| IBIS file stm32u535_545_ufbga64_smps.ibs
[IBIS ver] 4.2
[File name] stm32u535_545_ufbga64_smps.ibs
[File Rev] ev1.0
[Date]  11-09-2023
[Source] Data Created at STMicroelectronics
[Notes]  File originated from ELDO simulations.
[Disclaimer]  This information is for modeling purpose only and is
   not guaranteed. The information is subject to change without
   notice.
[Copyright] Copyright 2023 STMicroelectronics Inc.
|   Component stm32u535_545_ufbga64_smps
[Component] stm32u535_545_ufbga64_smps
[Manufacturer] STMicroelectronics
[Package]
| variable   typ   min   max
R_pkg  0  NA  NA
L_pkg  0  NA  NA
C_pkg  0  NA  NA
[Pin]   signal_name   model_name
A1  VDD  power
A2  VDD11  nc
A3  PH3-BOOT0  io8_100m_ft
A4  PB6  io8_100m_i2c_ft
A5  PB3  io8_100m_i2c_ft
A6  PD2  io8_100m_hslv_ft
A7  PC10  io8_100m_hslv_ft
A8  VDD  power
B1  VBAT  power
B2  VSS  gnd
B3  PC13  io8_100m_ft_v33
B4  PB4  io8_100m_i2c_ft
B5  PC11  io8_100m_hslv_ft
B6  PC12  io8_166m_hslv_ft
B7  VSS  gnd
B8  VDDUSB  power
C1  PC14-OSC32_IN   io8_100m_tamp_ft
C2  PC15-OSC32_OUT   io8_100m_tamp_ft
C3  PB8  io8_100m_hslv_i2c_ft
C4  PA15  io8_100m_ft
C5  PA14  io8_100m_ft
C6  PA13  io8_100m_ft
C7  PA12  io8_usb_ft
C8  PA11  io8_usb_ft
D1  PH0-OSC_IN  io8_100m_ft
D2  PH1-OSC_OUT  io8_100m_ft
D3  PB7  io8_166m_hslv_i2c_ft
D4  PB5  io8_166m_hslv_ft
D5  PA10  io8_100m_ft
D6  PA9  io8_100m_ft
D7  PA8  io8_166m_hslv_ft
D8  PC9  io8_100m_hslv_ft
E1  NRST  nc
E2  PC0  io8_100m_hslv_i2c_ft
E3  PC1  io8_166m_hslv_i2c_ft
E4  PC2  io8_100m_hslv_ft
E5  PA0  io8_100m_hslv_tamp_ft
E6  PB14  io8_100m_i2c_ft
E7  PC7  io8_100m_hslv_ft
E8  PC8  io8_100m_hslv_ft
F1  VSSA  nc
F2  PC3  io8_100m_hslv_ft
F3  PA1  io8_100m_hslv_tamp_ft
F4  PA4  io8_100m_hslv_ft
F5  PA6  io8_100m_hslv_ft
F6  PB10  io8_166m_hslv_i2c_ft
F7  PB15  io8_100m_ft
F8  PC6  io8_100m_hslv_ft
G1  VDDA  power
G2  PA2  io8_100m_hslv_ft
G3  PA5  io8_100m_ft
G4  PB2  io8_100m_hslv_tamp_ft
G5  PB1  io8_100m_hslv_ft
G6  VSSSMPS  nc
G7  VSS  gnd
G8  PB13  io8_100m_i2c_ft
H1  VDD  power
H2  PA3  io8_166m_hslv_ft
H3  PA7  io8_100m_hslv_i2c_ft
H4  PB0  io8_100m_hslv_ft
H5  VLXSMPS  nc
H6  VDDSMPS  nc
H7  VDD11  nc
H8  VDD  power
[Package Model]   455-ufbga-5x5-64smps-100mhz-230421
[Pin Mapping]   pulldown_ref   pullup_ref   | Comment
A1  nc  vddiom
A2  nc  nc
A3  gndio  vddiom
A4  gndio  vddiom
A5  gndio  vddiom
A6  gndio  vddiom
A7  gndio  vddiom
A8  nc  vddiom
B1  nc  vsw
B2  gndio  nc
B3  gndio  vddiom  | Depending on IO usage
| B3  gndio  vsw  | Depending on IO usage
B4  gndio  vddiom
B5  gndio  vddiom
B6  gndio  vddiom
B7  gndio  nc
B8  nc  vddusb
C1  gndio  vddiom  | Depending on IO usage
| C1  gndio  vsw  | Depending on IO usage
C2  gndio  vddiom  | Depending on IO usage
| C2  gndio  vsw  | Depending on IO usage
C3  gndio  vddiom
C4  gndio  vddiom
C5  gndio  vddiom
C6  gndio  vddiom  | Depending on IO usage
| C6  gndio  vddusb  | Depending on IO usage
C7  gndio  vddiom  | Depending on IO usage
| C7  gndio  vddusb  | Depending on IO usage
C8  gndio  vddiom  | Depending on IO usage
| C8  gndio  vddusb  | Depending on IO usage
D1  gndio  vddiom
D2  gndio  vddiom
D3  gndio  vddiom
D4  gndio  vddiom
D5  gndio  vddiom  | Depending on IO usage
| D5  gndio  vddusb  | Depending on IO usage
D6  gndio  vddiom  | Depending on IO usage
| D6  gndio  vddusb  | Depending on IO usage
D7  gndio  vddiom
D8  gndio  vddiom
E1  nc   nc
E2  gndio  vddiom
E3  gndio  vddiom
E4  gndio  vddiom
E5  gndio  vddiom
E6  gndio  vddiom
E7  gndio  vddiom
E8  gndio  vddiom
F1  nc  nc
F2  gndio  vddiom
F3  gndio  vddiom
F4  gndio  vddiom
F5  gndio  vddiom
F6  gndio  vddiom
F7  gndio  vddiom
F8  gndio  vddiom
G1  nc  vddiom
G2  gndio  vddiom
G3  gndio  vddiom
G4  gndio  vddiom
G5  gndio  vddiom
G6  nc  nc
G7  gndio  nc
G8  gndio  vddiom
H1  nc  vddiom
H2  gndio  vddiom
H3  gndio  vddiom
H4  gndio  vddiom
H5  nc  nc
H6  nc  nc
H7  nc  nc
H8  nc  vddiom
[Model Selector] io8_100m_ft
io8_100m_ft_hs_1v2  "IO8_FT 100MHz high speed @ 1.2V"
io8_100m_ft_fs_1v2  "IO8_FT 100MHz fast speed @ 1.2V"
io8_100m_ft_fs_pd_1v2  "IO8_FT 100MHz fast speed @ 1.2V pulldown"
io8_100m_ft_ms_1v2  "IO8_FT 100MHz med speed @ 1.2V"
io8_100m_ft_ms_pd_1v2  "IO8_FT 100MHz med speed @ 1.2V pulldown"
io8_100m_ft_ls_1v2  "IO8_FT 100MHz low speed @ 1.2V"
io8_100m_ft_ls_pd_1v2  "IO8_FT 100MHz low speed @ 1.2V pulldown"
io8_100m_ft_hs_1v8  "IO8_FT 100MHz high speed @ 1.8V"
io8_100m_ft_hs_pd_1v8  "IO8_FT 100MHz high speed @ 1.8V pulldown"
io8_100m_ft_fs_1v8  "IO8_FT 100MHz fast speed @ 1.8V"
io8_100m_ft_fs_pd_1v8  "IO8_FT 100MHz fast speed @ 1.8V pulldown"
io8_100m_ft_ms_1v8  "IO8_FT 100MHz med speed @ 1.8V"
io8_100m_ft_ms_pd_1v8  "IO8_FT 100MHz med speed @ 1.8V pulldown"
io8_100m_ft_ls_1v8  "IO8_FT 100MHz low speed @ 1.8V"
io8_100m_ft_ls_pd_1v8  "IO8_FT 100MHz low speed @ 1.8V pulldown"
io8_100m_ft_hs_3v3  "IO8_FT 100MHz high speed @ 3.3V"
io8_100m_ft_hs_pd_3v3  "IO8_FT 100MHz high speed @ 3.3V pulldown"
io8_100m_ft_fs_3v3  "IO8_FT 100MHz fast speed @ 3.3V"
io8_100m_ft_fs_pd_3v3  "IO8_FT 100MHz fast speed @ 3.3V pulldown"
io8_100m_ft_ms_3v3  "IO8_FT 100MHz med speed @ 3.3V"
io8_100m_ft_ms_pd_3v3  "IO8_FT 100MHz med speed @ 3.3V pulldown"
io8_100m_ft_ls_3v3  "IO8_FT 100MHz low speed @ 3.3V"
io8_100m_ft_ls_pd_3v3  "IO8_FT 100MHz low speed @ 3.3V pulldown"
[Model Selector] io8_100m_hslv_ft
io8_100m_ft_hs_1v2  "IO8_FT 100MHz high speed @ 1.2V"
io8_100m_ft_hs_pu_1v2  "IO8_FT 100MHz high speed @ 1.2V pullup"
io8_100m_ft_hs_pd_1v2  "IO8_FT 100MHz high speed @ 1.2V pulldown"
io8_100m_ft_fs_1v2  "IO8_FT 100MHz fast speed @ 1.2V"
io8_100m_ft_fs_pu_1v2  "IO8_FT 100MHz fast speed @ 1.2V pullup"
io8_100m_ft_fs_pd_1v2  "IO8_FT 100MHz fast speed @ 1.2V pulldown"
io8_100m_ft_ms_1v2  "IO8_FT 100MHz med speed @ 1.2V"
io8_100m_ft_ms_pu_1v2  "IO8_FT 100MHz med speed @ 1.2V pullup"
io8_100m_ft_ms_pd_1v2  "IO8_FT 100MHz med speed @ 1.2V pulldown"
io8_100m_ft_ls_1v2  "IO8_FT 100MHz low speed @ 1.2V"
io8_100m_ft_ls_pu_1v2  "IO8_FT 100MHz low speed @ 1.2V pullup"
io8_100m_ft_ls_pd_1v2  "IO8_FT 100MHz low speed @ 1.2V pulldown"
io8_100m_ft_hs_1v8  "IO8_FT 100MHz high speed @ 1.8V"
io8_100m_ft_hs_pu_1v8  "IO8_FT 100MHz high speed @ 1.8V pullup"
io8_100m_ft_hs_pd_1v8  "IO8_FT 100MHz high speed @ 1.8V pulldown"
io8_100m_ft_fs_1v8  "IO8_FT 100MHz fast speed @ 1.8V"
io8_100m_ft_fs_pu_1v8  "IO8_FT 100MHz fast speed @ 1.8V pullup"
io8_100m_ft_fs_pd_1v8  "IO8_FT 100MHz fast speed @ 1.8V pulldown"
io8_100m_ft_ms_1v8  "IO8_FT 100MHz med speed @ 1.8V"
io8_100m_ft_ms_pu_1v8  "IO8_FT 100MHz med speed @ 1.8V pullup"
io8_100m_ft_ms_pd_1v8  "IO8_FT 100MHz med speed @ 1.8V pulldown"
io8_100m_ft_ls_1v8  "IO8_FT 100MHz low speed @ 1.8V"
io8_100m_ft_ls_pu_1v8  "IO8_FT 100MHz low speed @ 1.8V pullup"
io8_100m_ft_ls_pd_1v8  "IO8_FT 100MHz low speed @ 1.8V pulldown"
io8_100m_ft_hs_3v3  "IO8_FT 100MHz high speed @ 3.3V"
io8_100m_ft_hs_pu_3v3  "IO8_FT 100MHz high speed @ 3.3V pullup"
io8_100m_ft_hs_pd_3v3  "IO8_FT 100MHz high speed @ 3.3V pulldown"
io8_100m_ft_fs_3v3  "IO8_FT 100MHz fast speed @ 3.3V"
io8_100m_ft_fs_pu_3v3  "IO8_FT 100MHz fast speed @ 3.3V pullup"
io8_100m_ft_fs_pd_3v3  "IO8_FT 100MHz fast speed @ 3.3V pulldown"
io8_100m_ft_ms_3v3  "IO8_FT 100MHz med speed @ 3.3V"
io8_100m_ft_ms_pu_3v3  "IO8_FT 100MHz med speed @ 3.3V pullup"
io8_100m_ft_ms_pd_3v3  "IO8_FT 100MHz med speed @ 3.3V pulldown"
io8_100m_ft_ls_3v3  "IO8_FT 100MHz low speed @ 3.3V"
io8_100m_ft_ls_pu_3v3  "IO8_FT 100MHz low speed @ 3.3V pullup"
io8_100m_ft_ls_pd_3v3  "IO8_FT 100MHz low speed @ 3.3V pulldown"
io8_100m_hslv_ft_hs_1v2  "IO8_FT 100MHz HSLV high speed @ 1.2V"
io8_100m_hslv_ft_hs_pu_1v2  "IO8_FT 100MHz HSLV high speed @ 1.2V pullup"
io8_100m_hslv_ft_hs_pd_1v2  "IO8_FT 100MHz HSLV high speed @ 1.2V pulldown"
io8_100m_hslv_ft_fs_1v2  "IO8_FT 100MHz HSLV fast speed @ 1.2V"
io8_100m_hslv_ft_fs_pu_1v2  "IO8_FT 100MHz HSLV fast speed @ 1.2V pullup"
io8_100m_hslv_ft_fs_pd_1v2  "IO8_FT 100MHz HSLV fast speed @ 1.2V pulldown"
io8_100m_hslv_ft_ms_1v2  "IO8_FT 100MHz HSLV med speed @ 1.2V"
io8_100m_hslv_ft_ms_pu_1v2  "IO8_FT 100MHz HSLV med speed @ 1.2V pullup"
io8_100m_hslv_ft_ms_pd_1v2  "IO8_FT 100MHz HSLV med speed @ 1.2V pulldown"
io8_100m_hslv_ft_ls_1v2  "IO8_FT 100MHz HSLV low speed @ 1.2V"
io8_100m_hslv_ft_ls_pu_1v2  "IO8_FT 100MHz HSLV low speed @ 1.2V pullup"
io8_100m_hslv_ft_ls_pd_1v2  "IO8_FT 100MHz HSLV low speed @ 1.2V pulldown"
io8_100m_hslv_ft_hs_1v8  "IO8_FT 100MHz HSLV high speed @ 1.8V"
io8_100m_hslv_ft_hs_pu_1v8  "IO8_FT 100MHz HSLV high speed @ 1.8V pullup"
io8_100m_hslv_ft_hs_pd_1v8  "IO8_FT 100MHz HSLV high speed @ 1.8V pulldown"
io8_100m_hslv_ft_fs_1v8  "IO8_FT 100MHz HSLV fast speed @ 1.8V"
io8_100m_hslv_ft_fs_pu_1v8  "IO8_FT 100MHz HSLV fast speed @ 1.8V pullup"
io8_100m_hslv_ft_fs_pd_1v8  "IO8_FT 100MHz HSLV fast speed @ 1.8V pulldown"
io8_100m_hslv_ft_ms_1v8  "IO8_FT 100MHz HSLV med speed @ 1.8V"
io8_100m_hslv_ft_ms_pu_1v8  "IO8_FT 100MHz HSLV med speed @ 1.8V pullup"
io8_100m_hslv_ft_ms_pd_1v8  "IO8_FT 100MHz HSLV med speed @ 1.8V pulldown"
io8_100m_hslv_ft_ls_1v8  "IO8_FT 100MHz HSLV low speed @ 1.8V"
io8_100m_hslv_ft_ls_pu_1v8  "IO8_FT 100MHz HSLV low speed @ 1.8V pullup"
io8_100m_hslv_ft_ls_pd_1v8  "IO8_FT 100MHz HSLV low speed @ 1.8V pulldown"
io8_100m_hslv_ft_hs_2v5  "IO8_FT 100MHz HSLV high speed @ 2.5V"
io8_100m_hslv_ft_hs_pu_2v5  "IO8_FT 100MHz HSLV high speed @ 2.5V pullup"
io8_100m_hslv_ft_hs_pd_2v5  "IO8_FT 100MHz HSLV high speed @ 2.5V pulldown"
io8_100m_hslv_ft_fs_2v5  "IO8_FT 100MHz HSLV fast speed @ 2.5V"
io8_100m_hslv_ft_fs_pu_2v5  "IO8_FT 100MHz HSLV fast speed @ 2.5V pullup"
io8_100m_hslv_ft_fs_pd_2v5  "IO8_FT 100MHz HSLV fast speed @ 2.5V pulldown"
io8_100m_hslv_ft_ms_2v5  "IO8_FT 100MHz HSLV med speed @ 2.5V"
io8_100m_hslv_ft_ms_pu_2v5  "IO8_FT 100MHz HSLV med speed @ 2.5V pullup"
io8_100m_hslv_ft_ms_pd_2v5  "IO8_FT 100MHz HSLV med speed @ 2.5V pulldown"
io8_100m_hslv_ft_ls_2v5  "IO8_FT 100MHz HSLV low speed @ 2.5V"
io8_100m_hslv_ft_ls_pu_2v5  "IO8_FT 100MHz HSLV low speed @ 2.5V pullup"
io8_100m_hslv_ft_ls_pd_2v5  "IO8_FT 100MHz HSLV low speed @ 2.5V pulldown"
[Model Selector] io8_100m_hslv_i2c_ft
io8_100m_ft_hs_1v2  "IO8_FT 100MHz high speed @ 1.2V"
io8_100m_ft_hs_pu_1v2  "IO8_FT 100MHz high speed @ 1.2V pullup"
io8_100m_ft_hs_pd_1v2  "IO8_FT 100MHz high speed @ 1.2V pulldown"
io8_100m_ft_fs_1v2  "IO8_FT 100MHz fast speed @ 1.2V"
io8_100m_ft_fs_pu_1v2  "IO8_FT 100MHz fast speed @ 1.2V pullup"
io8_100m_ft_fs_pd_1v2  "IO8_FT 100MHz fast speed @ 1.2V pulldown"
io8_100m_ft_ms_1v2  "IO8_FT 100MHz med speed @ 1.2V"
io8_100m_ft_ms_pu_1v2  "IO8_FT 100MHz med speed @ 1.2V pullup"
io8_100m_ft_ms_pd_1v2  "IO8_FT 100MHz med speed @ 1.2V pulldown"
io8_100m_ft_ls_1v2  "IO8_FT 100MHz low speed @ 1.2V"
io8_100m_ft_ls_pu_1v2  "IO8_FT 100MHz low speed @ 1.2V pullup"
io8_100m_ft_ls_pd_1v2  "IO8_FT 100MHz low speed @ 1.2V pulldown"
io8_100m_ft_hs_1v8  "IO8_FT 100MHz high speed @ 1.8V"
io8_100m_ft_hs_pu_1v8  "IO8_FT 100MHz high speed @ 1.8V pullup"
io8_100m_ft_hs_pd_1v8  "IO8_FT 100MHz high speed @ 1.8V pulldown"
io8_100m_ft_fs_1v8  "IO8_FT 100MHz fast speed @ 1.8V"
io8_100m_ft_fs_pu_1v8  "IO8_FT 100MHz fast speed @ 1.8V pullup"
io8_100m_ft_fs_pd_1v8  "IO8_FT 100MHz fast speed @ 1.8V pulldown"
io8_100m_ft_ms_1v8  "IO8_FT 100MHz med speed @ 1.8V"
io8_100m_ft_ms_pu_1v8  "IO8_FT 100MHz med speed @ 1.8V pullup"
io8_100m_ft_ms_pd_1v8  "IO8_FT 100MHz med speed @ 1.8V pulldown"
io8_100m_ft_ls_1v8  "IO8_FT 100MHz low speed @ 1.8V"
io8_100m_ft_ls_pu_1v8  "IO8_FT 100MHz low speed @ 1.8V pullup"
io8_100m_ft_ls_pd_1v8  "IO8_FT 100MHz low speed @ 1.8V pulldown"
io8_100m_ft_hs_3v3  "IO8_FT 100MHz high speed @ 3.3V"
io8_100m_ft_hs_pu_3v3  "IO8_FT 100MHz high speed @ 3.3V pullup"
io8_100m_ft_hs_pd_3v3  "IO8_FT 100MHz high speed @ 3.3V pulldown"
io8_100m_ft_fs_3v3  "IO8_FT 100MHz fast speed @ 3.3V"
io8_100m_ft_fs_pu_3v3  "IO8_FT 100MHz fast speed @ 3.3V pullup"
io8_100m_ft_fs_pd_3v3  "IO8_FT 100MHz fast speed @ 3.3V pulldown"
io8_100m_ft_ms_3v3  "IO8_FT 100MHz med speed @ 3.3V"
io8_100m_ft_ms_pu_3v3  "IO8_FT 100MHz med speed @ 3.3V pullup"
io8_100m_ft_ms_pd_3v3  "IO8_FT 100MHz med speed @ 3.3V pulldown"
io8_100m_ft_ls_3v3  "IO8_FT 100MHz low speed @ 3.3V"
io8_100m_ft_ls_pu_3v3  "IO8_FT 100MHz low speed @ 3.3V pullup"
io8_100m_ft_ls_pd_3v3  "IO8_FT 100MHz low speed @ 3.3V pulldown"
io8_100m_hslv_ft_hs_1v2  "IO8_FT 100MHz HSLV high speed @ 1.2V"
io8_100m_hslv_ft_hs_pu_1v2  "IO8_FT 100MHz HSLV high speed @ 1.2V pullup"
io8_100m_hslv_ft_hs_pd_1v2  "IO8_FT 100MHz HSLV high speed @ 1.2V pulldown"
io8_100m_hslv_ft_fs_1v2  "IO8_FT 100MHz HSLV fast speed @ 1.2V"
io8_100m_hslv_ft_fs_pu_1v2  "IO8_FT 100MHz HSLV fast speed @ 1.2V pullup"
io8_100m_hslv_ft_fs_pd_1v2  "IO8_FT 100MHz HSLV fast speed @ 1.2V pulldown"
io8_100m_hslv_ft_ms_1v2  "IO8_FT 100MHz HSLV med speed @ 1.2V"
io8_100m_hslv_ft_ms_pu_1v2  "IO8_FT 100MHz HSLV med speed @ 1.2V pullup"
io8_100m_hslv_ft_ms_pd_1v2  "IO8_FT 100MHz HSLV med speed @ 1.2V pulldown"
io8_100m_hslv_ft_ls_1v2  "IO8_FT 100MHz HSLV low speed @ 1.2V"
io8_100m_hslv_ft_ls_pu_1v2  "IO8_FT 100MHz HSLV low speed @ 1.2V pullup"
io8_100m_hslv_ft_ls_pd_1v2  "IO8_FT 100MHz HSLV low speed @ 1.2V pulldown"
io8_100m_hslv_ft_hs_1v8  "IO8_FT 100MHz HSLV high speed @ 1.8V"
io8_100m_hslv_ft_hs_pu_1v8  "IO8_FT 100MHz HSLV high speed @ 1.8V pullup"
io8_100m_hslv_ft_hs_pd_1v8  "IO8_FT 100MHz HSLV high speed @ 1.8V pulldown"
io8_100m_hslv_ft_fs_1v8  "IO8_FT 100MHz HSLV fast speed @ 1.8V"
io8_100m_hslv_ft_fs_pu_1v8  "IO8_FT 100MHz HSLV fast speed @ 1.8V pullup"
io8_100m_hslv_ft_fs_pd_1v8  "IO8_FT 100MHz HSLV fast speed @ 1.8V pulldown"
io8_100m_hslv_ft_ms_1v8  "IO8_FT 100MHz HSLV med speed @ 1.8V"
io8_100m_hslv_ft_ms_pu_1v8  "IO8_FT 100MHz HSLV med speed @ 1.8V pullup"
io8_100m_hslv_ft_ms_pd_1v8  "IO8_FT 100MHz HSLV med speed @ 1.8V pulldown"
io8_100m_hslv_ft_ls_1v8  "IO8_FT 100MHz HSLV low speed @ 1.8V"
io8_100m_hslv_ft_ls_pu_1v8  "IO8_FT 100MHz HSLV low speed @ 1.8V pullup"
io8_100m_hslv_ft_ls_pd_1v8  "IO8_FT 100MHz HSLV low speed @ 1.8V pulldown"
io8_100m_hslv_ft_hs_2v5  "IO8_FT 100MHz HSLV high speed @ 2.5V"
io8_100m_hslv_ft_hs_pu_2v5  "IO8_FT 100MHz HSLV high speed @ 2.5V pullup"
io8_100m_hslv_ft_hs_pd_2v5  "IO8_FT 100MHz HSLV high speed @ 2.5V pulldown"
io8_100m_hslv_ft_fs_2v5  "IO8_FT 100MHz HSLV fast speed @ 2.5V"
io8_100m_hslv_ft_fs_pu_2v5  "IO8_FT 100MHz HSLV fast speed @ 2.5V pullup"
io8_100m_hslv_ft_fs_pd_2v5  "IO8_FT 100MHz HSLV fast speed @ 2.5V pulldown"
io8_100m_hslv_ft_ms_2v5  "IO8_FT 100MHz HSLV med speed @ 2.5V"
io8_100m_hslv_ft_ms_pu_2v5  "IO8_FT 100MHz HSLV med speed @ 2.5V pullup"
io8_100m_hslv_ft_ms_pd_2v5  "IO8_FT 100MHz HSLV med speed @ 2.5V pulldown"
io8_100m_hslv_ft_ls_2v5  "IO8_FT 100MHz HSLV low speed @ 2.5V"
io8_100m_hslv_ft_ls_pu_2v5  "IO8_FT 100MHz HSLV low speed @ 2.5V pullup"
io8_100m_hslv_ft_ls_pd_2v5  "IO8_FT 100MHz HSLV low speed @ 2.5V pulldown"
[Model Selector] io8_100m_hslv_tamp_ft
io8_100m_ft_hs_1v2  "IO8_FT 100MHz high speed @ 1.2V"
io8_100m_ft_hs_pu_1v2  "IO8_FT 100MHz high speed @ 1.2V pullup"
io8_100m_ft_hs_pd_1v2  "IO8_FT 100MHz high speed @ 1.2V pulldown"
io8_100m_ft_fs_1v2  "IO8_FT 100MHz fast speed @ 1.2V"
io8_100m_ft_fs_pu_1v2  "IO8_FT 100MHz fast speed @ 1.2V pullup"
io8_100m_ft_fs_pd_1v2  "IO8_FT 100MHz fast speed @ 1.2V pulldown"
io8_100m_ft_ms_1v2  "IO8_FT 100MHz med speed @ 1.2V"
io8_100m_ft_ms_pu_1v2  "IO8_FT 100MHz med speed @ 1.2V pullup"
io8_100m_ft_ms_pd_1v2  "IO8_FT 100MHz med speed @ 1.2V pulldown"
io8_100m_ft_ls_1v2  "IO8_FT 100MHz low speed @ 1.2V"
io8_100m_ft_ls_pu_1v2  "IO8_FT 100MHz low speed @ 1.2V pullup"
io8_100m_ft_ls_pd_1v2  "IO8_FT 100MHz low speed @ 1.2V pulldown"
io8_100m_ft_hs_1v8  "IO8_FT 100MHz high speed @ 1.8V"
io8_100m_ft_hs_pu_1v8  "IO8_FT 100MHz high speed @ 1.8V pullup"
io8_100m_ft_hs_pd_1v8  "IO8_FT 100MHz high speed @ 1.8V pulldown"
io8_100m_ft_fs_1v8  "IO8_FT 100MHz fast speed @ 1.8V"
io8_100m_ft_fs_pu_1v8  "IO8_FT 100MHz fast speed @ 1.8V pullup"
io8_100m_ft_fs_pd_1v8  "IO8_FT 100MHz fast speed @ 1.8V pulldown"
io8_100m_ft_ms_1v8  "IO8_FT 100MHz med speed @ 1.8V"
io8_100m_ft_ms_pu_1v8  "IO8_FT 100MHz med speed @ 1.8V pullup"
io8_100m_ft_ms_pd_1v8  "IO8_FT 100MHz med speed @ 1.8V pulldown"
io8_100m_ft_ls_1v8  "IO8_FT 100MHz low speed @ 1.8V"
io8_100m_ft_ls_pu_1v8  "IO8_FT 100MHz low speed @ 1.8V pullup"
io8_100m_ft_ls_pd_1v8  "IO8_FT 100MHz low speed @ 1.8V pulldown"
io8_100m_ft_hs_3v3  "IO8_FT 100MHz high speed @ 3.3V"
io8_100m_ft_hs_pu_3v3  "IO8_FT 100MHz high speed @ 3.3V pullup"
io8_100m_ft_hs_pd_3v3  "IO8_FT 100MHz high speed @ 3.3V pulldown"
io8_100m_ft_fs_3v3  "IO8_FT 100MHz fast speed @ 3.3V"
io8_100m_ft_fs_pu_3v3  "IO8_FT 100MHz fast speed @ 3.3V pullup"
io8_100m_ft_fs_pd_3v3  "IO8_FT 100MHz fast speed @ 3.3V pulldown"
io8_100m_ft_ms_3v3  "IO8_FT 100MHz med speed @ 3.3V"
io8_100m_ft_ms_pu_3v3  "IO8_FT 100MHz med speed @ 3.3V pullup"
io8_100m_ft_ms_pd_3v3  "IO8_FT 100MHz med speed @ 3.3V pulldown"
io8_100m_ft_ls_3v3  "IO8_FT 100MHz low speed @ 3.3V"
io8_100m_ft_ls_pu_3v3  "IO8_FT 100MHz low speed @ 3.3V pullup"
io8_100m_ft_ls_pd_3v3  "IO8_FT 100MHz low speed @ 3.3V pulldown"
io8_100m_hslv_ft_hs_1v2  "IO8_FT 100MHz HSLV high speed @ 1.2V"
io8_100m_hslv_ft_hs_pu_1v2  "IO8_FT 100MHz HSLV high speed @ 1.2V pullup"
io8_100m_hslv_ft_hs_pd_1v2  "IO8_FT 100MHz HSLV high speed @ 1.2V pulldown"
io8_100m_hslv_ft_fs_1v2  "IO8_FT 100MHz HSLV fast speed @ 1.2V"
io8_100m_hslv_ft_fs_pu_1v2  "IO8_FT 100MHz HSLV fast speed @ 1.2V pullup"
io8_100m_hslv_ft_fs_pd_1v2  "IO8_FT 100MHz HSLV fast speed @ 1.2V pulldown"
io8_100m_hslv_ft_ms_1v2  "IO8_FT 100MHz HSLV med speed @ 1.2V"
io8_100m_hslv_ft_ms_pu_1v2  "IO8_FT 100MHz HSLV med speed @ 1.2V pullup"
io8_100m_hslv_ft_ms_pd_1v2  "IO8_FT 100MHz HSLV med speed @ 1.2V pulldown"
io8_100m_hslv_ft_ls_1v2  "IO8_FT 100MHz HSLV low speed @ 1.2V"
io8_100m_hslv_ft_ls_pu_1v2  "IO8_FT 100MHz HSLV low speed @ 1.2V pullup"
io8_100m_hslv_ft_ls_pd_1v2  "IO8_FT 100MHz HSLV low speed @ 1.2V pulldown"
io8_100m_hslv_ft_hs_1v8  "IO8_FT 100MHz HSLV high speed @ 1.8V"
io8_100m_hslv_ft_hs_pu_1v8  "IO8_FT 100MHz HSLV high speed @ 1.8V pullup"
io8_100m_hslv_ft_hs_pd_1v8  "IO8_FT 100MHz HSLV high speed @ 1.8V pulldown"
io8_100m_hslv_ft_fs_1v8  "IO8_FT 100MHz HSLV fast speed @ 1.8V"
io8_100m_hslv_ft_fs_pu_1v8  "IO8_FT 100MHz HSLV fast speed @ 1.8V pullup"
io8_100m_hslv_ft_fs_pd_1v8  "IO8_FT 100MHz HSLV fast speed @ 1.8V pulldown"
io8_100m_hslv_ft_ms_1v8  "IO8_FT 100MHz HSLV med speed @ 1.8V"
io8_100m_hslv_ft_ms_pu_1v8  "IO8_FT 100MHz HSLV med speed @ 1.8V pullup"
io8_100m_hslv_ft_ms_pd_1v8  "IO8_FT 100MHz HSLV med speed @ 1.8V pulldown"
io8_100m_hslv_ft_ls_1v8  "IO8_FT 100MHz HSLV low speed @ 1.8V"
io8_100m_hslv_ft_ls_pu_1v8  "IO8_FT 100MHz HSLV low speed @ 1.8V pullup"
io8_100m_hslv_ft_ls_pd_1v8  "IO8_FT 100MHz HSLV low speed @ 1.8V pulldown"
io8_100m_hslv_ft_hs_2v5  "IO8_FT 100MHz HSLV high speed @ 2.5V"
io8_100m_hslv_ft_hs_pu_2v5  "IO8_FT 100MHz HSLV high speed @ 2.5V pullup"
io8_100m_hslv_ft_hs_pd_2v5  "IO8_FT 100MHz HSLV high speed @ 2.5V pulldown"
io8_100m_hslv_ft_fs_2v5  "IO8_FT 100MHz HSLV fast speed @ 2.5V"
io8_100m_hslv_ft_fs_pu_2v5  "IO8_FT 100MHz HSLV fast speed @ 2.5V pullup"
io8_100m_hslv_ft_fs_pd_2v5  "IO8_FT 100MHz HSLV fast speed @ 2.5V pulldown"
io8_100m_hslv_ft_ms_2v5  "IO8_FT 100MHz HSLV med speed @ 2.5V"
io8_100m_hslv_ft_ms_pu_2v5  "IO8_FT 100MHz HSLV med speed @ 2.5V pullup"
io8_100m_hslv_ft_ms_pd_2v5  "IO8_FT 100MHz HSLV med speed @ 2.5V pulldown"
io8_100m_hslv_ft_ls_2v5  "IO8_FT 100MHz HSLV low speed @ 2.5V"
io8_100m_hslv_ft_ls_pu_2v5  "IO8_FT 100MHz HSLV low speed @ 2.5V pullup"
io8_100m_hslv_ft_ls_pd_2v5  "IO8_FT 100MHz HSLV low speed @ 2.5V pulldown"
io8_ft_v33_hs_1v2  "IO8_FT_V33 high speed @ 1.2V"
io8_ft_v33_hs_pu_1v2  "IO8_FT_V33 high speed @ 1.2V pullup"
io8_ft_v33_hs_pd_1v2  "IO8_FT_V33 high speed @ 1.2V pulldown"
io8_ft_v33_fs_1v2  "IO8_FT_V33 fast speed @ 1.2V"
io8_ft_v33_fs_pu_1v2  "IO8_FT_V33 fast speed @ 1.2V pullup"
io8_ft_v33_fs_pd_1v2  "IO8_FT_V33 fast speed @ 1.2V pulldown"
io8_ft_v33_ms_1v2  "IO8_FT_V33 med speed @ 1.2V"
io8_ft_v33_ms_pu_1v2  "IO8_FT_V33 med speed @ 1.2V pullup"
io8_ft_v33_ms_pd_1v2  "IO8_FT_V33 med speed @ 1.2V pulldown"
io8_ft_v33_ls_1v2  "IO8_FT_V33 low speed @ 1.2V"
io8_ft_v33_ls_pu_1v2  "IO8_FT_V33 low speed @ 1.2V pullup"
io8_ft_v33_ls_pd_1v2  "IO8_FT_V33 low speed @ 1.2V pulldown"
io8_ft_v33_hs_1v8  "IO8_FT_V33 high speed @ 1.8V"
io8_ft_v33_hs_pu_1v8  "IO8_FT_V33 high speed @ 1.8V pullup"
io8_ft_v33_hs_pd_1v8  "IO8_FT_V33 high speed @ 1.8V pulldown"
io8_ft_v33_fs_1v8  "IO8_FT_V33 fast speed @ 1.8V"
io8_ft_v33_fs_pu_1v8  "IO8_FT_V33 fast speed @ 1.8V pullup"
io8_ft_v33_fs_pd_1v8  "IO8_FT_V33 fast speed @ 1.8V pulldown"
io8_ft_v33_ms_1v8  "IO8_FT_V33 med speed @ 1.8V"
io8_ft_v33_ms_pu_1v8  "IO8_FT_V33 med speed @ 1.8V pullup"
io8_ft_v33_ms_pd_1v8  "IO8_FT_V33 med speed @ 1.8V pulldown"
io8_ft_v33_ls_1v8  "IO8_FT_V33 low speed @ 1.8V"
io8_ft_v33_ls_pu_1v8  "IO8_FT_V33 low speed @ 1.8V pullup"
io8_ft_v33_ls_pd_1v8  "IO8_FT_V33 low speed @ 1.8V pulldown"
io8_ft_v33_hs_3v3  "IO8_FT_V33 high speed @ 3.3V"
io8_ft_v33_hs_pu_3v3  "IO8_FT_V33 high speed @ 3.3V pullup"
io8_ft_v33_hs_pd_3v3  "IO8_FT_V33 high speed @ 3.3V pulldown"
io8_ft_v33_fs_3v3  "IO8_FT_V33 fast speed @ 3.3V"
io8_ft_v33_fs_pu_3v3  "IO8_FT_V33 fast speed @ 3.3V pullup"
io8_ft_v33_fs_pd_3v3  "IO8_FT_V33 fast speed @ 3.3V pulldown"
io8_ft_v33_ms_3v3  "IO8_FT_V33 med speed @ 3.3V"
io8_ft_v33_ms_pu_3v3  "IO8_FT_V33 med speed @ 3.3V pullup"
io8_ft_v33_ms_pd_3v3  "IO8_FT_V33 med speed @ 3.3V pulldown"
io8_ft_v33_ls_3v3  "IO8_FT_V33 low speed @ 3.3V"
io8_ft_v33_ls_pu_3v3  "IO8_FT_V33 low speed @ 3.3V pullup"
io8_ft_v33_ls_pd_3v3  "IO8_FT_V33 low speed @ 3.3V pulldown"
[Model Selector] io8_100m_i2c_ft
io8_100m_ft_hs_1v2  "IO8_FT 100MHz high speed @ 1.2V"
io8_100m_ft_hs_pu_1v2  "IO8_FT 100MHz high speed @ 1.2V pullup"
io8_100m_ft_hs_pd_1v2  "IO8_FT 100MHz high speed @ 1.2V pulldown"
io8_100m_ft_fs_1v2  "IO8_FT 100MHz fast speed @ 1.2V"
io8_100m_ft_fs_pu_1v2  "IO8_FT 100MHz fast speed @ 1.2V pullup"
io8_100m_ft_fs_pd_1v2  "IO8_FT 100MHz fast speed @ 1.2V pulldown"
io8_100m_ft_ms_1v2  "IO8_FT 100MHz med speed @ 1.2V"
io8_100m_ft_ms_pu_1v2  "IO8_FT 100MHz med speed @ 1.2V pullup"
io8_100m_ft_ms_pd_1v2  "IO8_FT 100MHz med speed @ 1.2V pulldown"
io8_100m_ft_ls_1v2  "IO8_FT 100MHz low speed @ 1.2V"
io8_100m_ft_ls_pu_1v2  "IO8_FT 100MHz low speed @ 1.2V pullup"
io8_100m_ft_ls_pd_1v2  "IO8_FT 100MHz low speed @ 1.2V pulldown"
io8_100m_ft_hs_1v8  "IO8_FT 100MHz high speed @ 1.8V"
io8_100m_ft_hs_pu_1v8  "IO8_FT 100MHz high speed @ 1.8V pullup"
io8_100m_ft_hs_pd_1v8  "IO8_FT 100MHz high speed @ 1.8V pulldown"
io8_100m_ft_fs_1v8  "IO8_FT 100MHz fast speed @ 1.8V"
io8_100m_ft_fs_pu_1v8  "IO8_FT 100MHz fast speed @ 1.8V pullup"
io8_100m_ft_fs_pd_1v8  "IO8_FT 100MHz fast speed @ 1.8V pulldown"
io8_100m_ft_ms_1v8  "IO8_FT 100MHz med speed @ 1.8V"
io8_100m_ft_ms_pu_1v8  "IO8_FT 100MHz med speed @ 1.8V pullup"
io8_100m_ft_ms_pd_1v8  "IO8_FT 100MHz med speed @ 1.8V pulldown"
io8_100m_ft_ls_1v8  "IO8_FT 100MHz low speed @ 1.8V"
io8_100m_ft_ls_pu_1v8  "IO8_FT 100MHz low speed @ 1.8V pullup"
io8_100m_ft_ls_pd_1v8  "IO8_FT 100MHz low speed @ 1.8V pulldown"
io8_100m_ft_hs_3v3  "IO8_FT 100MHz high speed @ 3.3V"
io8_100m_ft_hs_pu_3v3  "IO8_FT 100MHz high speed @ 3.3V pullup"
io8_100m_ft_hs_pd_3v3  "IO8_FT 100MHz high speed @ 3.3V pulldown"
io8_100m_ft_fs_3v3  "IO8_FT 100MHz fast speed @ 3.3V"
io8_100m_ft_fs_pu_3v3  "IO8_FT 100MHz fast speed @ 3.3V pullup"
io8_100m_ft_fs_pd_3v3  "IO8_FT 100MHz fast speed @ 3.3V pulldown"
io8_100m_ft_ms_3v3  "IO8_FT 100MHz med speed @ 3.3V"
io8_100m_ft_ms_pu_3v3  "IO8_FT 100MHz med speed @ 3.3V pullup"
io8_100m_ft_ms_pd_3v3  "IO8_FT 100MHz med speed @ 3.3V pulldown"
io8_100m_ft_ls_3v3  "IO8_FT 100MHz low speed @ 3.3V"
io8_100m_ft_ls_pu_3v3  "IO8_FT 100MHz low speed @ 3.3V pullup"
io8_100m_ft_ls_pd_3v3  "IO8_FT 100MHz low speed @ 3.3V pulldown"
io8_100m_i2c_ft_1v2  "IO8_FT 100MHz I2C @ 1.2V"
io8_100m_i2c_ft_pu_1v2  "IO8_FT 100MHz I2C @ 1.2V pullup"
io8_100m_i2c_ft_pd_1v2  "IO8_FT 100MHz I2C @ 1.2V pulldown"
io8_100m_i2c_ft_1v8  "IO8_FT 100MHz I2C @ 1.8V"
io8_100m_i2c_ft_pu_1v8  "IO8_FT 100MHz I2C @ 1.8V pullup"
io8_100m_i2c_ft_pd_1v8  "IO8_FT 100MHz I2C @ 1,8V pulldown"
io8_100m_i2c_ft_3v3  "IO8_FT 100MHz I2C @ 3.3V"
io8_100m_i2c_ft_pu_3v3  "IO8_FT 100MHz I2C HSLV @ 3.3V pullup"
io8_100m_i2c_ft_pd_3v3  "IO8_FT 100MHz I2C @ 3.3V pulldown"
[Model Selector] io8_100m_tamp_ft
io8_100m_ft_hs_1v2  "IO8_FT 100MHz high speed @ 1.2V"
io8_100m_ft_hs_pu_1v2  "IO8_FT 100MHz high speed @ 1.2V pullup"
io8_100m_ft_hs_pd_1v2  "IO8_FT 100MHz high speed @ 1.2V pulldown"
io8_100m_ft_fs_1v2  "IO8_FT 100MHz fast speed @ 1.2V"
io8_100m_ft_fs_pu_1v2  "IO8_FT 100MHz fast speed @ 1.2V pullup"
io8_100m_ft_fs_pd_1v2  "IO8_FT 100MHz fast speed @ 1.2V pulldown"
io8_100m_ft_ms_1v2  "IO8_FT 100MHz med speed @ 1.2V"
io8_100m_ft_ms_pu_1v2  "IO8_FT 100MHz med speed @ 1.2V pullup"
io8_100m_ft_ms_pd_1v2  "IO8_FT 100MHz med speed @ 1.2V pulldown"
io8_100m_ft_ls_1v2  "IO8_FT 100MHz low speed @ 1.2V"
io8_100m_ft_ls_pu_1v2  "IO8_FT 100MHz low speed @ 1.2V pullup"
io8_100m_ft_ls_pd_1v2  "IO8_FT 100MHz low speed @ 1.2V pulldown"
io8_100m_ft_hs_1v8  "IO8_FT 100MHz high speed @ 1.8V"
io8_100m_ft_hs_pu_1v8  "IO8_FT 100MHz high speed @ 1.8V pullup"
io8_100m_ft_hs_pd_1v8  "IO8_FT 100MHz high speed @ 1.8V pulldown"
io8_100m_ft_fs_1v8  "IO8_FT 100MHz fast speed @ 1.8V"
io8_100m_ft_fs_pu_1v8  "IO8_FT 100MHz fast speed @ 1.8V pullup"
io8_100m_ft_fs_pd_1v8  "IO8_FT 100MHz fast speed @ 1.8V pulldown"
io8_100m_ft_ms_1v8  "IO8_FT 100MHz med speed @ 1.8V"
io8_100m_ft_ms_pu_1v8  "IO8_FT 100MHz med speed @ 1.8V pullup"
io8_100m_ft_ms_pd_1v8  "IO8_FT 100MHz med speed @ 1.8V pulldown"
io8_100m_ft_ls_1v8  "IO8_FT 100MHz low speed @ 1.8V"
io8_100m_ft_ls_pu_1v8  "IO8_FT 100MHz low speed @ 1.8V pullup"
io8_100m_ft_ls_pd_1v8  "IO8_FT 100MHz low speed @ 1.8V pulldown"
io8_100m_ft_hs_3v3  "IO8_FT 100MHz high speed @ 3.3V"
io8_100m_ft_hs_pu_3v3  "IO8_FT 100MHz high speed @ 3.3V pullup"
io8_100m_ft_hs_pd_3v3  "IO8_FT 100MHz high speed @ 3.3V pulldown"
io8_100m_ft_fs_3v3  "IO8_FT 100MHz fast speed @ 3.3V"
io8_100m_ft_fs_pu_3v3  "IO8_FT 100MHz fast speed @ 3.3V pullup"
io8_100m_ft_fs_pd_3v3  "IO8_FT 100MHz fast speed @ 3.3V pulldown"
io8_100m_ft_ms_3v3  "IO8_FT 100MHz med speed @ 3.3V"
io8_100m_ft_ms_pu_3v3  "IO8_FT 100MHz med speed @ 3.3V pullup"
io8_100m_ft_ms_pd_3v3  "IO8_FT 100MHz med speed @ 3.3V pulldown"
io8_100m_ft_ls_3v3  "IO8_FT 100MHz low speed @ 3.3V"
io8_100m_ft_ls_pu_3v3  "IO8_FT 100MHz low speed @ 3.3V pullup"
io8_100m_ft_ls_pd_3v3  "IO8_FT 100MHz low speed @ 3.3V pulldown"
io8_ft_v33_hs_1v2  "IO8_FT_V33 high speed @ 1.2V"
io8_ft_v33_hs_pu_1v2  "IO8_FT_V33 high speed @ 1.2V pullup"
io8_ft_v33_hs_pd_1v2  "IO8_FT_V33 high speed @ 1.2V pulldown"
io8_ft_v33_fs_1v2  "IO8_FT_V33 fast speed @ 1.2V"
io8_ft_v33_fs_pu_1v2  "IO8_FT_V33 fast speed @ 1.2V pullup"
io8_ft_v33_fs_pd_1v2  "IO8_FT_V33 fast speed @ 1.2V pulldown"
io8_ft_v33_ms_1v2  "IO8_FT_V33 med speed @ 1.2V"
io8_ft_v33_ms_pu_1v2  "IO8_FT_V33 med speed @ 1.2V pullup"
io8_ft_v33_ms_pd_1v2  "IO8_FT_V33 med speed @ 1.2V pulldown"
io8_ft_v33_ls_1v2  "IO8_FT_V33 low speed @ 1.2V"
io8_ft_v33_ls_pu_1v2  "IO8_FT_V33 low speed @ 1.2V pullup"
io8_ft_v33_ls_pd_1v2  "IO8_FT_V33 low speed @ 1.2V pulldown"
io8_ft_v33_hs_1v8  "IO8_FT_V33 high speed @ 1.8V"
io8_ft_v33_hs_pu_1v8  "IO8_FT_V33 high speed @ 1.8V pullup"
io8_ft_v33_hs_pd_1v8  "IO8_FT_V33 high speed @ 1.8V pulldown"
io8_ft_v33_fs_1v8  "IO8_FT_V33 fast speed @ 1.8V"
io8_ft_v33_fs_pu_1v8  "IO8_FT_V33 fast speed @ 1.8V pullup"
io8_ft_v33_fs_pd_1v8  "IO8_FT_V33 fast speed @ 1.8V pulldown"
io8_ft_v33_ms_1v8  "IO8_FT_V33 med speed @ 1.8V"
io8_ft_v33_ms_pu_1v8  "IO8_FT_V33 med speed @ 1.8V pullup"
io8_ft_v33_ms_pd_1v8  "IO8_FT_V33 med speed @ 1.8V pulldown"
io8_ft_v33_ls_1v8  "IO8_FT_V33 low speed @ 1.8V"
io8_ft_v33_ls_pu_1v8  "IO8_FT_V33 low speed @ 1.8V pullup"
io8_ft_v33_ls_pd_1v8  "IO8_FT_V33 low speed @ 1.8V pulldown"
io8_ft_v33_hs_3v3  "IO8_FT_V33 high speed @ 3.3V"
io8_ft_v33_hs_pu_3v3  "IO8_FT_V33 high speed @ 3.3V pullup"
io8_ft_v33_hs_pd_3v3  "IO8_FT_V33 high speed @ 3.3V pulldown"
io8_ft_v33_fs_3v3  "IO8_FT_V33 fast speed @ 3.3V"
io8_ft_v33_fs_pu_3v3  "IO8_FT_V33 fast speed @ 3.3V pullup"
io8_ft_v33_fs_pd_3v3  "IO8_FT_V33 fast speed @ 3.3V pulldown"
io8_ft_v33_ms_3v3  "IO8_FT_V33 med speed @ 3.3V"
io8_ft_v33_ms_pu_3v3  "IO8_FT_V33 med speed @ 3.3V pullup"
io8_ft_v33_ms_pd_3v3  "IO8_FT_V33 med speed @ 3.3V pulldown"
io8_ft_v33_ls_3v3  "IO8_FT_V33 low speed @ 3.3V"
io8_ft_v33_ls_pu_3v3  "IO8_FT_V33 low speed @ 3.3V pullup"
io8_ft_v33_ls_pd_3v3  "IO8_FT_V33 low speed @ 3.3V pulldown"
[Model Selector] io8_usb_ft
io8_100m_ft_hs_1v2  "IO8_FT 100MHz high speed @ 1.2V"
io8_100m_ft_hs_pu_1v2  "IO8_FT 100MHz high speed @ 1.2V pullup"
io8_100m_ft_hs_pd_1v2  "IO8_FT 100MHz high speed @ 1.2V pulldown"
io8_100m_ft_fs_1v2  "IO8_FT 100MHz fast speed @ 1.2V"
io8_100m_ft_fs_pu_1v2  "IO8_FT 100MHz fast speed @ 1.2V pullup"
io8_100m_ft_fs_pd_1v2  "IO8_FT 100MHz fast speed @ 1.2V pulldown"
io8_100m_ft_ms_1v2  "IO8_FT 100MHz med speed @ 1.2V"
io8_100m_ft_ms_pu_1v2  "IO8_FT 100MHz med speed @ 1.2V pullup"
io8_100m_ft_ms_pd_1v2  "IO8_FT 100MHz med speed @ 1.2V pulldown"
io8_100m_ft_ls_1v2  "IO8_FT 100MHz low speed @ 1.2V"
io8_100m_ft_ls_pu_1v2  "IO8_FT 100MHz low speed @ 1.2V pullup"
io8_100m_ft_ls_pd_1v2  "IO8_FT 100MHz low speed @ 1.2V pulldown"
io8_100m_ft_hs_1v8  "IO8_FT 100MHz high speed @ 1.8V"
io8_100m_ft_hs_pu_1v8  "IO8_FT 100MHz high speed @ 1.8V pullup"
io8_100m_ft_hs_pd_1v8  "IO8_FT 100MHz high speed @ 1.8V pulldown"
io8_100m_ft_fs_1v8  "IO8_FT 100MHz fast speed @ 1.8V"
io8_100m_ft_fs_pu_1v8  "IO8_FT 100MHz fast speed @ 1.8V pullup"
io8_100m_ft_fs_pd_1v8  "IO8_FT 100MHz fast speed @ 1.8V pulldown"
io8_100m_ft_ms_1v8  "IO8_FT 100MHz med speed @ 1.8V"
io8_100m_ft_ms_pu_1v8  "IO8_FT 100MHz med speed @ 1.8V pullup"
io8_100m_ft_ms_pd_1v8  "IO8_FT 100MHz med speed @ 1.8V pulldown"
io8_100m_ft_ls_1v8  "IO8_FT 100MHz low speed @ 1.8V"
io8_100m_ft_ls_pu_1v8  "IO8_FT 100MHz low speed @ 1.8V pullup"
io8_100m_ft_ls_pd_1v8  "IO8_FT 100MHz low speed @ 1.8V pulldown"
io8_100m_ft_hs_3v3  "IO8_FT 100MHz high speed @ 3.3V"
io8_100m_ft_hs_pu_3v3  "IO8_FT 100MHz high speed @ 3.3V pullup"
io8_100m_ft_hs_pd_3v3  "IO8_FT 100MHz high speed @ 3.3V pulldown"
io8_100m_ft_fs_3v3  "IO8_FT 100MHz fast speed @ 3.3V"
io8_100m_ft_fs_pu_3v3  "IO8_FT 100MHz fast speed @ 3.3V pullup"
io8_100m_ft_fs_pd_3v3  "IO8_FT 100MHz fast speed @ 3.3V pulldown"
io8_100m_ft_ms_3v3  "IO8_FT 100MHz med speed @ 3.3V"
io8_100m_ft_ms_pu_3v3  "IO8_FT 100MHz med speed @ 3.3V pullup"
io8_100m_ft_ms_pd_3v3  "IO8_FT 100MHz med speed @ 3.3V pulldown"
io8_100m_ft_ls_3v3  "IO8_FT 100MHz low speed @ 3.3V"
io8_100m_ft_ls_pu_3v3  "IO8_FT 100MHz low speed @ 3.3V pullup"
io8_100m_ft_ls_pd_3v3  "IO8_FT 100MHz low speed @ 3.3V pulldown"
io8_usb_fs_3v3  "IOUSB fast speed @ 3.3V"
io8_usb_fs_pu1_3v3  "IO8USB fast speed @ 3.3V pullup1"
io8_usb_fs_pd1_3v3  "IOUSB fast speed @ 3.3V pulldown1"
io8_usb_ls_3v3  "IOUSB low speed @ 3.3V"
io8_usb_ls_pu1_3v3  "IOUSB low speed @ 3.3V pullup1"
io8_usb_ls_pd1_3v3  "IOUSB low speed @ 3.3V pulldown1"
io8_usb_fs_pu2_3v3  "IOUSB fast speed @ 3.3V pullup2"
io8_usb_fs_pd2_3v3  "IOUSB fast speed @ 3.3V pulldown2"
io8_usb_ls_pu2_3v3  "IOUSB low speed @ 3.3V pullup2"
io8_usb_ls_pd2_3v3  "IOUSB low speed @ 3.3V pulldown2"
[Model Selector] io8_166m_hslv_ft
io8_166m_ft_hs_1v2  "IO8_FT 166MHz high speed @ 1.2V"
io8_166m_ft_hs_pu_1v2  "IO8_FT 166MHz high speed @ 1.2V pullup"
io8_166m_ft_hs_pd_1v2  "IO8_FT 166MHz high speed @ 1.2V pulldown"
io8_166m_ft_fs_1v2  "IO8_FT 166MHz fast speed @ 1.2V"
io8_166m_ft_fs_pu_1v2  "IO8_FT 166MHz fast speed @ 1.2V pullup"
io8_166m_ft_fs_pd_1v2  "IO8_FT 166MHz fast speed @ 1.2V pulldown"
io8_166m_ft_ms_1v2  "IO8_FT 166MHz med speed @ 1.2V"
io8_166m_ft_ms_pu_1v2  "IO8_FT 166MHz med speed @ 1.2V pullup"
io8_166m_ft_ms_pd_1v2  "IO8_FT 166MHz med speed @ 1.2V pulldown"
io8_166m_ft_ls_1v2  "IO8_FT 166MHz low speed @ 1.2V"
io8_166m_ft_ls_pu_1v2  "IO8_FT 166MHz low speed @ 1.2V pullup"
io8_166m_ft_ls_pd_1v2  "IO8_FT 166MHz low speed @ 1.2V pulldown"
io8_166m_ft_hs_1v8  "IO8_FT 166MHz high speed @ 1.8V"
io8_166m_ft_hs_pu_1v8  "IO8_FT 166MHz high speed @ 1.8V pullup"
io8_166m_ft_hs_pd_1v8  "IO8_FT 166MHz high speed @ 1.8V pulldown"
io8_166m_ft_fs_1v8  "IO8_FT 166MHz fast speed @ 1.8V"
io8_166m_ft_fs_pu_1v8  "IO8_FT 166MHz fast speed @ 1.8V pullup"
io8_166m_ft_fs_pd_1v8  "IO8_FT 166MHz fast speed @ 1.8V pulldown"
io8_166m_ft_ms_1v8  "IO8_FT 166MHz med speed @ 1.8V"
io8_166m_ft_ms_pu_1v8  "IO8_FT 166MHz med speed @ 1.8V pullup"
io8_166m_ft_ms_pd_1v8  "IO8_FT 166MHz med speed @ 1.8V pulldown"
io8_166m_ft_ls_1v8  "IO8_FT 166MHz low speed @ 1.8V"
io8_166m_ft_ls_pu_1v8  "IO8_FT 166MHz low speed @ 1.8V pullup"
io8_166m_ft_ls_pd_1v8  "IO8_FT 166MHz low speed @ 1.8V pulldown"
io8_166m_ft_hs_3v3  "IO8_FT 166MHz high speed @ 3.3V"
io8_166m_ft_hs_pu_3v3  "IO8_FT 166MHz high speed @ 3.3V pullup"
io8_166m_ft_hs_pd_3v3  "IO8_FT 166MHz high speed @ 3.3V pulldown"
io8_166m_ft_fs_3v3  "IO8_FT 166MHz fast speed @ 3.3V"
io8_166m_ft_fs_pu_3v3  "IO8_FT 166MHz fast speed @ 3.3V pullup"
io8_166m_ft_fs_pd_3v3  "IO8_FT 166MHz fast speed @ 3.3V pulldown"
io8_166m_ft_ms_3v3  "IO8_FT 166MHz med speed @ 3.3V"
io8_166m_ft_ms_pu_3v3  "IO8_FT 166MHz med speed @ 3.3V pullup"
io8_166m_ft_ms_pd_3v3  "IO8_FT 166MHz med speed @ 3.3V pulldown"
io8_166m_ft_ls_3v3  "IO8_FT 166MHz low speed @ 3.3V"
io8_166m_ft_ls_pu_3v3  "IO8_FT 166MHz low speed @ 3.3V pullup"
io8_166m_ft_ls_pd_3v3  "IO8_FT 166MHz low speed @ 3.3V pulldown"
io8_166m_hslv_ft_hs_1v2  "IO8_FT 166MHz HSLV high speed @ 1.2V"
io8_166m_hslv_ft_hs_pu_1v2  "IO8_FT 166MHz HSLV high speed @ 1.2V pullup"
io8_166m_hslv_ft_hs_pd_1v2  "IO8_FT 166MHz HSLV high speed @ 1.2V pulldown"
io8_166m_hslv_ft_fs_1v2  "IO8_FT 166MHz HSLV fast speed @ 1.2V"
io8_166m_hslv_ft_fs_pu_1v2  "IO8_FT 166MHz HSLV fast speed @ 1.2V pullup"
io8_166m_hslv_ft_fs_pd_1v2  "IO8_FT 166MHz HSLV fast speed @ 1.2V pulldown"
io8_166m_hslv_ft_ms_1v2  "IO8_FT 166MHz HSLV med speed @ 1.2V"
io8_166m_hslv_ft_ms_pu_1v2  "IO8_FT 166MHz HSLV med speed @ 1.2V pullup"
io8_166m_hslv_ft_ms_pd_1v2  "IO8_FT 166MHz HSLV med speed @ 1.2V pulldown"
io8_166m_hslv_ft_ls_1v2  "IO8_FT 166MHz HSLV low speed @ 1.2V"
io8_166m_hslv_ft_ls_pu_1v2  "IO8_FT 166MHz HSLV low speed @ 1.2V pullup"
io8_166m_hslv_ft_ls_pd_1v2  "IO8_FT 166MHz HSLV low speed @ 1.2V pulldown"
io8_166m_hslv_ft_hs_1v8  "IO8_FT 166MHz HSLV high speed @ 1.8V"
io8_166m_hslv_ft_hs_pu_1v8  "IO8_FT 166MHz HSLV high speed @ 1.8V pullup"
io8_166m_hslv_ft_hs_pd_1v8  "IO8_FT 166MHz HSLV high speed @ 1.8V pulldown"
io8_166m_hslv_ft_fs_1v8  "IO8_FT 166MHz HSLV fast speed @ 1.8V"
io8_166m_hslv_ft_fs_pu_1v8  "IO8_FT 166MHz HSLV fast speed @ 1.8V pullup"
io8_166m_hslv_ft_fs_pd_1v8  "IO8_FT 166MHz HSLV fast speed @ 1.8V pulldown"
io8_166m_hslv_ft_ms_1v8  "IO8_FT 166MHz HSLV med speed @ 1.8V"
io8_166m_hslv_ft_ms_pu_1v8  "IO8_FT 166MHz HSLV med speed @ 1.8V pullup"
io8_166m_hslv_ft_ms_pd_1v8  "IO8_FT 166MHz HSLV med speed @ 1.8V pulldown"
io8_166m_hslv_ft_ls_1v8  "IO8_FT 166MHz HSLV low speed @ 1.8V"
io8_166m_hslv_ft_ls_pu_1v8  "IO8_FT 166MHz HSLV low speed @ 1.8V pullup"
io8_166m_hslv_ft_ls_pd_1v8  "IO8_FT 166MHz HSLV low speed @ 1.8V pulldown"
io8_166m_hslv_ft_hs_2v5  "IO8_FT 166MHz HSLV high speed @ 2.5V"
io8_166m_hslv_ft_hs_pu_2v5  "IO8_FT 166MHz HSLV high speed @ 2.5V pullup"
io8_166m_hslv_ft_hs_pd_2v5  "IO8_FT 166MHz HSLV high speed @ 2.5V pulldown"
io8_166m_hslv_ft_fs_2v5  "IO8_FT 166MHz HSLV fast speed @ 2.5V"
io8_166m_hslv_ft_fs_pu_2v5  "IO8_FT 166MHz HSLV fast speed @ 2.5V pullup"
io8_166m_hslv_ft_fs_pd_2v5  "IO8_FT 166MHz HSLV fast speed @ 2.5V pulldown"
io8_166m_hslv_ft_ms_2v5  "IO8_FT 166MHz HSLV med speed @ 2.5V"
io8_166m_hslv_ft_ms_pu_2v5  "IO8_FT 166MHz HSLV med speed @ 2.5V pullup"
io8_166m_hslv_ft_ms_pd_2v5  "IO8_FT 166MHz HSLV med speed @ 2.5V pulldown"
io8_166m_hslv_ft_ls_2v5  "IO8_FT 166MHz HSLV low speed @ 2.5V"
io8_166m_hslv_ft_ls_pu_2v5  "IO8_FT 166MHz HSLV low speed @ 2.5V pullup"
io8_166m_hslv_ft_ls_pd_2v5  "IO8_FT 166MHz HSLV low speed @ 2.5V pulldown"
[Model Selector] io8_166m_hslv_i2c_ft
io8_166m_ft_hs_1v2  "IO8_FT 166MHz high speed @ 1.2V"
io8_166m_ft_hs_pu_1v2  "IO8_FT 166MHz high speed @ 1.2V pullup"
io8_166m_ft_hs_pd_1v2  "IO8_FT 166MHz high speed @ 1.2V pulldown"
io8_166m_ft_fs_1v2  "IO8_FT 166MHz fast speed @ 1.2V"
io8_166m_ft_fs_pu_1v2  "IO8_FT 166MHz fast speed @ 1.2V pullup"
io8_166m_ft_fs_pd_1v2  "IO8_FT 166MHz fast speed @ 1.2V pulldown"
io8_166m_ft_ms_1v2  "IO8_FT 166MHz med speed @ 1.2V"
io8_166m_ft_ms_pu_1v2  "IO8_FT 166MHz med speed @ 1.2V pullup"
io8_166m_ft_ms_pd_1v2  "IO8_FT 166MHz med speed @ 1.2V pulldown"
io8_166m_ft_ls_1v2  "IO8_FT 166MHz low speed @ 1.2V"
io8_166m_ft_ls_pu_1v2  "IO8_FT 166MHz low speed @ 1.2V pullup"
io8_166m_ft_ls_pd_1v2  "IO8_FT 166MHz low speed @ 1.2V pulldown"
io8_166m_ft_hs_1v8  "IO8_FT 166MHz high speed @ 1.8V"
io8_166m_ft_hs_pu_1v8  "IO8_FT 166MHz high speed @ 1.8V pullup"
io8_166m_ft_hs_pd_1v8  "IO8_FT 166MHz high speed @ 1.8V pulldown"
io8_166m_ft_fs_1v8  "IO8_FT 166MHz fast speed @ 1.8V"
io8_166m_ft_fs_pu_1v8  "IO8_FT 166MHz fast speed @ 1.8V pullup"
io8_166m_ft_fs_pd_1v8  "IO8_FT 166MHz fast speed @ 1.8V pulldown"
io8_166m_ft_ms_1v8  "IO8_FT 166MHz med speed @ 1.8V"
io8_166m_ft_ms_pu_1v8  "IO8_FT 166MHz med speed @ 1.8V pullup"
io8_166m_ft_ms_pd_1v8  "IO8_FT 166MHz med speed @ 1.8V pulldown"
io8_166m_ft_ls_1v8  "IO8_FT 166MHz low speed @ 1.8V"
io8_166m_ft_ls_pu_1v8  "IO8_FT 166MHz low speed @ 1.8V pullup"
io8_166m_ft_ls_pd_1v8  "IO8_FT 166MHz low speed @ 1.8V pulldown"
io8_166m_ft_hs_3v3  "IO8_FT 166MHz high speed @ 3.3V"
io8_166m_ft_hs_pu_3v3  "IO8_FT 166MHz high speed @ 3.3V pullup"
io8_166m_ft_hs_pd_3v3  "IO8_FT 166MHz high speed @ 3.3V pulldown"
io8_166m_ft_fs_3v3  "IO8_FT 166MHz fast speed @ 3.3V"
io8_166m_ft_fs_pu_3v3  "IO8_FT 166MHz fast speed @ 3.3V pullup"
io8_166m_ft_fs_pd_3v3  "IO8_FT 166MHz fast speed @ 3.3V pulldown"
io8_166m_ft_ms_3v3  "IO8_FT 166MHz med speed @ 3.3V"
io8_166m_ft_ms_pu_3v3  "IO8_FT 166MHz med speed @ 3.3V pullup"
io8_166m_ft_ms_pd_3v3  "IO8_FT 166MHz med speed @ 3.3V pulldown"
io8_166m_ft_ls_3v3  "IO8_FT 166MHz low speed @ 3.3V"
io8_166m_ft_ls_pu_3v3  "IO8_FT 166MHz low speed @ 3.3V pullup"
io8_166m_ft_ls_pd_3v3  "IO8_FT 166MHz low speed @ 3.3V pulldown"
io8_166m_hslv_ft_hs_1v2  "IO8_FT 166MHz HSLV high speed @ 1.2V"
io8_166m_hslv_ft_hs_pu_1v2  "IO8_FT 166MHz HSLV high speed @ 1.2V pullup"
io8_166m_hslv_ft_hs_pd_1v2  "IO8_FT 166MHz HSLV high speed @ 1.2V pulldown"
io8_166m_hslv_ft_fs_1v2  "IO8_FT 166MHz HSLV fast speed @ 1.2V"
io8_166m_hslv_ft_fs_pu_1v2  "IO8_FT 166MHz HSLV fast speed @ 1.2V pullup"
io8_166m_hslv_ft_fs_pd_1v2  "IO8_FT 166MHz HSLV fast speed @ 1.2V pulldown"
io8_166m_hslv_ft_ms_1v2  "IO8_FT 166MHz HSLV med speed @ 1.2V"
io8_166m_hslv_ft_ms_pu_1v2  "IO8_FT 166MHz HSLV med speed @ 1.2V pullup"
io8_166m_hslv_ft_ms_pd_1v2  "IO8_FT 166MHz HSLV med speed @ 1.2V pulldown"
io8_166m_hslv_ft_ls_1v2  "IO8_FT 166MHz HSLV low speed @ 1.2V"
io8_166m_hslv_ft_ls_pu_1v2  "IO8_FT 166MHz HSLV low speed @ 1.2V pullup"
io8_166m_hslv_ft_ls_pd_1v2  "IO8_FT 166MHz HSLV low speed @ 1.2V pulldown"
io8_166m_hslv_ft_hs_1v8  "IO8_FT 166MHz HSLV high speed @ 1.8V"
io8_166m_hslv_ft_hs_pu_1v8  "IO8_FT 166MHz HSLV high speed @ 1.8V pullup"
io8_166m_hslv_ft_hs_pd_1v8  "IO8_FT 166MHz HSLV high speed @ 1.8V pulldown"
io8_166m_hslv_ft_fs_1v8  "IO8_FT 166MHz HSLV fast speed @ 1.8V"
io8_166m_hslv_ft_fs_pu_1v8  "IO8_FT 166MHz HSLV fast speed @ 1.8V pullup"
io8_166m_hslv_ft_fs_pd_1v8  "IO8_FT 166MHz HSLV fast speed @ 1.8V pulldown"
io8_166m_hslv_ft_ms_1v8  "IO8_FT 166MHz HSLV med speed @ 1.8V"
io8_166m_hslv_ft_ms_pu_1v8  "IO8_FT 166MHz HSLV med speed @ 1.8V pullup"
io8_166m_hslv_ft_ms_pd_1v8  "IO8_FT 166MHz HSLV med speed @ 1.8V pulldown"
io8_166m_hslv_ft_ls_1v8  "IO8_FT 166MHz HSLV low speed @ 1.8V"
io8_166m_hslv_ft_ls_pu_1v8  "IO8_FT 166MHz HSLV low speed @ 1.8V pullup"
io8_166m_hslv_ft_ls_pd_1v8  "IO8_FT 166MHz HSLV low speed @ 1.8V pulldown"
io8_166m_hslv_ft_hs_2v5  "IO8_FT 166MHz HSLV high speed @ 2.5V"
io8_166m_hslv_ft_hs_pu_2v5  "IO8_FT 166MHz HSLV high speed @ 2.5V pullup"
io8_166m_hslv_ft_hs_pd_2v5  "IO8_FT 166MHz HSLV high speed @ 2.5V pulldown"
io8_166m_hslv_ft_fs_2v5  "IO8_FT 166MHz HSLV fast speed @ 2.5V"
io8_166m_hslv_ft_fs_pu_2v5  "IO8_FT 166MHz HSLV fast speed @ 2.5V pullup"
io8_166m_hslv_ft_fs_pd_2v5  "IO8_FT 166MHz HSLV fast speed @ 2.5V pulldown"
io8_166m_hslv_ft_ms_2v5  "IO8_FT 166MHz HSLV med speed @ 2.5V"
io8_166m_hslv_ft_ms_pu_2v5  "IO8_FT 166MHz HSLV med speed @ 2.5V pullup"
io8_166m_hslv_ft_ms_pd_2v5  "IO8_FT 166MHz HSLV med speed @ 2.5V pulldown"
io8_166m_hslv_ft_ls_2v5  "IO8_FT 166MHz HSLV low speed @ 2.5V"
io8_166m_hslv_ft_ls_pu_2v5  "IO8_FT 166MHz HSLV low speed @ 2.5V pullup"
io8_166m_hslv_ft_ls_pd_2v5  "IO8_FT 166MHz HSLV low speed @ 2.5V pulldown"
io8_166m_i2c_ft_1v2  "IO8_FT 166MHz I2C @ 1.2V"
io8_166m_i2c_ft_pu_1v2  "IO8_FT 166MHz I2C @ 1.2V pullup"
io8_166m_i2c_ft_pd_1v2  "IO8_FT 166MHz I2C @ 1.2V pulldown"
io8_166m_i2c_ft_1v8  "IO8_FT 166MHz I2C @ 1.8V"
io8_166m_i2c_ft_pu_1v8  "IO8_FT 166MHz I2C @ 1.8V pullup"
io8_166m_i2c_ft_pd_1v8  "IO8_FT 166MHz I2C @ 1,8V pulldown"
io8_166m_i2c_ft_3v3  "IO8_FT 166MHz I2C @ 3.3V"
io8_166m_i2c_ft_pu_3v3  "IO8_FT 166MHz I2C HSLV @ 3.3V pullup"
io8_166m_i2c_ft_pd_3v3  "IO8_FT 166MHz I2C @ 3.3V pulldown"
[Model Selector] io8_100m_ft_v33
io8_ft_v33_hs_1v2  "IO8_FT_V33 high speed @ 1.2V"
io8_ft_v33_hs_pu_1v2  "IO8_FT_V33 high speed @ 1.2V pullup"
io8_ft_v33_hs_pd_1v2  "IO8_FT_V33 high speed @ 1.2V pulldown"
io8_ft_v33_fs_1v2  "IO8_FT_V33 fast speed @ 1.2V"
io8_ft_v33_fs_pu_1v2  "IO8_FT_V33 fast speed @ 1.2V pullup"
io8_ft_v33_fs_pd_1v2  "IO8_FT_V33 fast speed @ 1.2V pulldown"
io8_ft_v33_ms_1v2  "IO8_FT_V33 med speed @ 1.2V"
io8_ft_v33_ms_pu_1v2  "IO8_FT_V33 med speed @ 1.2V pullup"
io8_ft_v33_ms_pd_1v2  "IO8_FT_V33 med speed @ 1.2V pulldown"
io8_ft_v33_ls_1v2  "IO8_FT_V33 low speed @ 1.2V"
io8_ft_v33_ls_pu_1v2  "IO8_FT_V33 low speed @ 1.2V pullup"
io8_ft_v33_ls_pd_1v2  "IO8_FT_V33 low speed @ 1.2V pulldown"
io8_ft_v33_hs_1v8  "IO8_FT_V33 high speed @ 1.8V"
io8_ft_v33_hs_pu_1v8  "IO8_FT_V33 high speed @ 1.8V pullup"
io8_ft_v33_hs_pd_1v8  "IO8_FT_V33 high speed @ 1.8V pulldown"
io8_ft_v33_fs_1v8  "IO8_FT_V33 fast speed @ 1.8V"
io8_ft_v33_fs_pu_1v8  "IO8_FT_V33 fast speed @ 1.8V pullup"
io8_ft_v33_fs_pd_1v8  "IO8_FT_V33 fast speed @ 1.8V pulldown"
io8_ft_v33_ms_1v8  "IO8_FT_V33 med speed @ 1.8V"
io8_ft_v33_ms_pu_1v8  "IO8_FT_V33 med speed @ 1.8V pullup"
io8_ft_v33_ms_pd_1v8  "IO8_FT_V33 med speed @ 1.8V pulldown"
io8_ft_v33_ls_1v8  "IO8_FT_V33 low speed @ 1.8V"
io8_ft_v33_ls_pu_1v8  "IO8_FT_V33 low speed @ 1.8V pullup"
io8_ft_v33_ls_pd_1v8  "IO8_FT_V33 low speed @ 1.8V pulldown"
io8_ft_v33_hs_3v3  "IO8_FT_V33 high speed @ 3.3V"
io8_ft_v33_hs_pu_3v3  "IO8_FT_V33 high speed @ 3.3V pullup"
io8_ft_v33_hs_pd_3v3  "IO8_FT_V33 high speed @ 3.3V pulldown"
io8_ft_v33_fs_3v3  "IO8_FT_V33 fast speed @ 3.3V"
io8_ft_v33_fs_pu_3v3  "IO8_FT_V33 fast speed @ 3.3V pullup"
io8_ft_v33_fs_pd_3v3  "IO8_FT_V33 fast speed @ 3.3V pulldown"
io8_ft_v33_ms_3v3  "IO8_FT_V33 med speed @ 3.3V"
io8_ft_v33_ms_pu_3v3  "IO8_FT_V33 med speed @ 3.3V pullup"
io8_ft_v33_ms_pd_3v3  "IO8_FT_V33 med speed @ 3.3V pulldown"
io8_ft_v33_ls_3v3  "IO8_FT_V33 low speed @ 3.3V"
io8_ft_v33_ls_pu_3v3  "IO8_FT_V33 low speed @ 3.3V pullup"
io8_ft_v33_ls_pd_3v3  "IO8_FT_V33 low speed @ 3.3V pulldown"
[Define Package Model]  455-ufbga-5x5-64smps-100mhz-230421
[Manufacturer]  unknown
[OEM]  unknown
[Description]  unknown
[Number Of Pins]  59
[Pin Numbers]
| Pin Name Terminal   Net Name   Starting Node   Ending Node
E1 | NRST
E5 | PA0
F3 | PA1
G2 | PA2
H2 | PA3
F4 | PA4
G3 | PA5
F5 | PA6
H3 | PA7
D7 | PA8
D6 | PA9
D5 | PA10
C8 | PA11
C7 | PA12
C6 | PA13
C5 | PA14
C4 | PA15
H4 | PB0
G5 | PB1
G4 | PB2
A5 | PB3
B4 | PB4
D4 | PB5
A4 | PB6
D3 | PB7
C3 | PB8
F6 | PB10
G8 | PB13
E6 | PB14
F7 | PB15
E2 | PC0
E3 | PC1
E4 | PC2
F2 | PC3
F8 | PC6
E7 | PC7
E8 | PC8
D8 | PC9
A7 | PC10
B5 | PC11
B6 | PC12
B3 | PC13
C1 | PC14-OSC32_IN
C2 | PC15-OSC32_OUT
A6 | PD2
D1 | PH0-OSC_IN
D2 | PH1-OSC_OUT
A3 | PH3-BOOT0
H7 | VDD11
A2 | VDD11
B1 | VBAT
A1 | VDD
G1 | VDDA
H6 | VDDSMPS
B8 | VDDUSB
H5 | VLXSMPS
B2 | VSS
F1 | VSSA
G6 | VSSSMPS
|[Merged Pins]  A1
|A8  |  VDD
|H1  |  VDD
|H8  |  VDD
|[Merged Pins]  B2
|B7  |  VSS
|G7  |  VSS
[Model Data]
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[End Model Data]
[End Package Model]
| Models and submodels in the file (208): io8_100m_ft_hs_1v2 (I/O), io8_100m_ft_hs_pu_1v2 (I/O), io8_100m_ft_hs_pd_1v2 (I/O), io8_100m_ft_fs_1v2 (I/O), io8_100m_ft_fs_pu_1v2 (I/O), io8_100m_ft_fs_pd_1v2 (I/O), io8_100m_ft_ms_1v2 (I/O), io8_100m_ft_ms_pu_1v2 (I/O), io8_100m_ft_ms_pd_1v2 (I/O), io8_100m_ft_ls_1v2 (I/O), io8_100m_ft_ls_pu_1v2 (I/O), io8_100m_ft_ls_pd_1v2 (I/O), io8_100m_ft_hs_1v8 (I/O), io8_100m_ft_hs_pu_1v8 (I/O), io8_100m_ft_hs_pd_1v8 (I/O), io8_100m_ft_fs_1v8 (I/O), io8_100m_ft_fs_pu_1v8 (I/O), io8_100m_ft_fs_pd_1v8 (I/O), io8_100m_ft_ms_1v8 (I/O), io8_100m_ft_ms_pu_1v8 (I/O), io8_100m_ft_ms_pd_1v8 (I/O), io8_100m_ft_ls_1v8 (I/O), io8_100m_ft_ls_pu_1v8 (I/O), io8_100m_ft_ls_pd_1v8 (I/O), io8_100m_ft_hs_3v3 (I/O), io8_100m_ft_hs_pu_3v3 (I/O), io8_100m_ft_hs_pd_3v3 (I/O), io8_100m_ft_fs_3v3 (I/O), io8_100m_ft_fs_pu_3v3 (I/O), io8_100m_ft_fs_pd_3v3 (I/O), io8_100m_ft_ms_3v3 (I/O), io8_100m_ft_ms_pu_3v3 (I/O), io8_100m_ft_ms_pd_3v3 (I/O), io8_100m_ft_ls_3v3 (I/O), io8_100m_ft_ls_pu_3v3 (I/O), io8_100m_ft_ls_pd_3v3 (I/O), io8_100m_hslv_ft_hs_1v2 (I/O), io8_100m_hslv_ft_hs_pu_1v2 (I/O), io8_100m_hslv_ft_hs_pd_1v2 (I/O), io8_100m_hslv_ft_fs_1v2 (I/O), io8_100m_hslv_ft_fs_pu_1v2 (I/O), io8_100m_hslv_ft_fs_pd_1v2 (I/O), io8_100m_hslv_ft_ms_1v2 (I/O), io8_100m_hslv_ft_ms_pu_1v2 (I/O), io8_100m_hslv_ft_ms_pd_1v2 (I/O), io8_100m_hslv_ft_ls_1v2 (I/O), io8_100m_hslv_ft_ls_pu_1v2 (I/O), io8_100m_hslv_ft_ls_pd_1v2 (I/O), io8_100m_hslv_ft_hs_1v8 (I/O), io8_100m_hslv_ft_hs_pu_1v8 (I/O), io8_100m_hslv_ft_hs_pd_1v8 (I/O), io8_100m_hslv_ft_fs_1v8 (I/O), io8_100m_hslv_ft_fs_pu_1v8 (I/O), io8_100m_hslv_ft_fs_pd_1v8 (I/O), io8_100m_hslv_ft_ms_1v8 (I/O), io8_100m_hslv_ft_ms_pu_1v8 (I/O), io8_100m_hslv_ft_ms_pd_1v8 (I/O), io8_100m_hslv_ft_ls_1v8 (I/O), io8_100m_hslv_ft_ls_pu_1v8 (I/O), io8_100m_hslv_ft_ls_pd_1v8 (I/O), io8_100m_hslv_ft_hs_2v5 (I/O), io8_100m_hslv_ft_hs_pu_2v5 (I/O), io8_100m_hslv_ft_hs_pd_2v5 (I/O), io8_100m_hslv_ft_fs_2v5 (I/O), io8_100m_hslv_ft_fs_pu_2v5 (I/O), io8_100m_hslv_ft_fs_pd_2v5 (I/O), io8_100m_hslv_ft_ms_2v5 (I/O), io8_100m_hslv_ft_ms_pu_2v5 (I/O), io8_100m_hslv_ft_ms_pd_2v5 (I/O), io8_100m_hslv_ft_ls_2v5 (I/O), io8_100m_hslv_ft_ls_pu_2v5 (I/O), io8_100m_hslv_ft_ls_pd_2v5 (I/O), io8_166m_ft_hs_1v2 (I/O), io8_166m_ft_hs_pu_1v2 (I/O), io8_166m_ft_hs_pd_1v2 (I/O), io8_166m_ft_fs_1v2 (I/O), io8_166m_ft_fs_pu_1v2 (I/O), io8_166m_ft_fs_pd_1v2 (I/O), io8_166m_ft_ms_1v2 (I/O), io8_166m_ft_ms_pu_1v2 (I/O)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
